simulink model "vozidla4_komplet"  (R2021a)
settings: Solver=VariableStepAuto  StartTime=0.0  StopTime=90  RelTol=1e-9
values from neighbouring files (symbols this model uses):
  A = A(1:(pocet_stavu),1:(pocet_stavu))    [appDekompLQR.m]    (also in appLQR.m = A(1:(2*N-1),1:(2*N-1)); appSYM.m = A(1:(2*N-1),1:(2*N-1)); appSZV.m = A(1:(2*N-1),1:(2*N-1)); central_LQR.m = A(1:(2*N-1),1:(2*N-1)))
  B = zeros(pocet_stavu,N)    [appDekompLQR.m]    (also in appLQR.m = zeros(2*N-1,N); appSYM.m = zeros(2*N-1,N); appSZV.m = zeros(2*N-1,N); central_LQR.m = zeros(2*N-1,N))
  C = eye(pocet_stavu)    [appDekompLQR.m]    (also in appLQR.m; appSYM.m; appSZV.m; central_LQR.m)
  conds0 = zeros(1,2*N-1)    [central_LQR.m]    (also in central_SYM.m; distri_STRUKTURAL.m = zeros(1,pocet_stavu); distri_SZV.m; porovnani_rizeni.m)
  D = zeros(pocet_stavu,N)    [appDekompLQR.m]    (also in appLQR.m; appSYM.m; appSZV.m; central_LQR.m)
  K = zeros(N,pocet_stavu)    [appDekompLQR.m]    (also in appSYM.m = [[0,-1/5,0,-3/20,0,-1/10,0,-1/20,0]; appSZV.m = [[-5/2,-3,7/4,1/2,0,0,0];[-1/7,-2/7,-7/2,-37/7,18/7,0,0];[0,; central_LQR.m = -K; central_SYM.m = [[0,-1/5,0,-3/20,0,-1/10,0,-1/20,0])

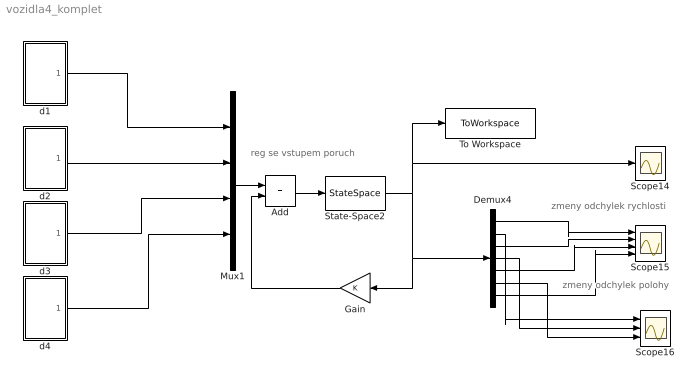
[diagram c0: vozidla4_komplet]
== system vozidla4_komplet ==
  note: zmeny odchylek polohy
  note: zmeny odchylek rychlosti
  note: reg se vstupem poruch
  Add : Sum
  Demux4 : Demux  Outputs=7
  Gain : Gain  Gain=K  Multiplication=Matrix(K*u)
  Mux1 : Mux
  Scope14 : Scope
  Scope15 : Scope  NumInputPorts=4
  Scope16 : Scope  NumInputPorts=3
  State-Space2 : StateSpace  A=A  B=B  C=C  D=D  InitialCondition=conds0
  To Workspace : ToWorkspace  VariableName=vystup  SaveFormat=Structure  SampleTime=-1
  d1 : Subsystem
  d2 : Subsystem
  d3 : Subsystem
  d4 : Subsystem
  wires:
  Demux4/6 -> Scope16/3
  Demux4/4 -> Scope16/2
  Demux4/7 -> Scope15/4
  Demux4/2 -> Scope16/1
  Demux4/3 -> Scope15/2
  Demux4/5 -> Scope15/3
  Demux4/1 -> Scope15/1
  Mux1/1 -> Add/1
  Gain/1 -> Add/2
  State-Space2/1 -> Demux4/1, Gain/1, Scope14/1, To Workspace/1
  Add/1 -> State-Space2/1
  d1/1(Out1) -> Mux1/1
  d4/1(Out1) -> Mux1/4
  d2/1(Out1) -> Mux1/2
  d3/1(Out1) -> Mux1/3

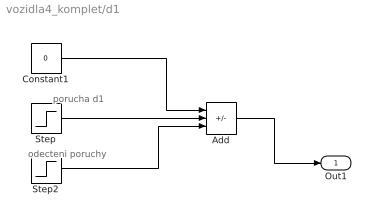
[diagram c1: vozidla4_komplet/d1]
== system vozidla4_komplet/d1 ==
  note: odecteni poruchy
  note: porucha d1
  Add : Sum  Inputs=++-
  Constant1 : Constant  Value=0
  Step : Step  Time=5  After=2  SampleTime=0
  Step2 : Step  Time=6  After=2  SampleTime=0
  Out1 : Outport
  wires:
  Constant1/1 -> Add/1
  Step2/1 -> Add/3
  Add/1 -> Out1/1
  Step/1 -> Add/2

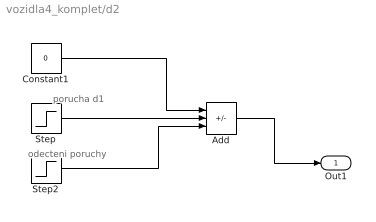
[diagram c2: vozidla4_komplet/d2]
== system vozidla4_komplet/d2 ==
  note: odecteni poruchy
  note: porucha d1
  Add : Sum  Inputs=++-
  Constant1 : Constant  Value=0
  Step : Step  Time=25  After=2  SampleTime=0
  Step2 : Step  Time=26  After=2  SampleTime=0
  Out1 : Outport
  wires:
  Constant1/1 -> Add/1
  Step2/1 -> Add/3
  Add/1 -> Out1/1
  Step/1 -> Add/2

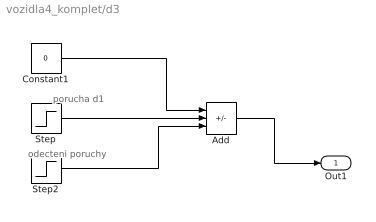
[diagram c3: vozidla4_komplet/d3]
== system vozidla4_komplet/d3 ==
  note: odecteni poruchy
  note: porucha d1
  Add : Sum  Inputs=++-
  Constant1 : Constant  Value=0
  Step : Step  Time=45  After=2  SampleTime=0
  Step2 : Step  Time=46  After=2  SampleTime=0
  Out1 : Outport
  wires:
  Constant1/1 -> Add/1
  Step2/1 -> Add/3
  Add/1 -> Out1/1
  Step/1 -> Add/2

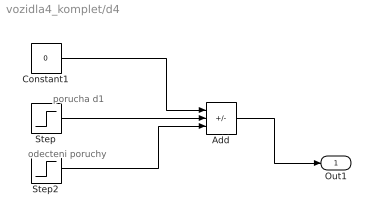
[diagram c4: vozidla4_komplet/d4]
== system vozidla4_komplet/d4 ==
  note: odecteni poruchy
  note: porucha d1
  Add : Sum  Inputs=++-
  Constant1 : Constant  Value=0
  Step : Step  Time=65  After=2  SampleTime=0
  Step2 : Step  Time=66  After=2  SampleTime=0
  Out1 : Outport
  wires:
  Constant1/1 -> Add/1
  Step2/1 -> Add/3
  Add/1 -> Out1/1
  Step/1 -> Add/2
